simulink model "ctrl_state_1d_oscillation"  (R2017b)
settings: Solver=ode45  StartTime=0.0  StopTime=60  RelTol=1e-3
undefined symbols (not defined in the file or in its folder): b
libraries: dps x8

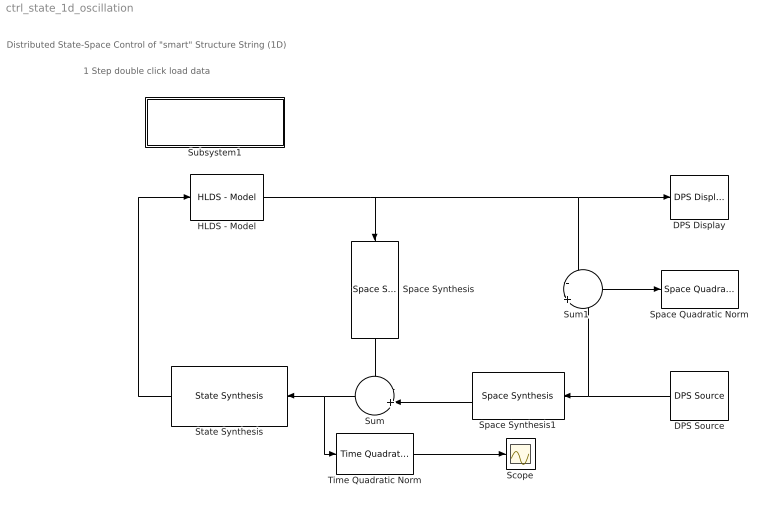
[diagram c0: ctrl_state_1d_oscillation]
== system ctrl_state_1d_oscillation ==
  note: Distributed State-Space Control of "smart" Structure String (1D)
  note: 1 Step double click load data
  DPS Display : dps/DPS Display  graphType=surf  pointCoord=[0:10]'  elementsVar=[1 2; 2 3; 3 4; 4 5; 5 6; 6 7; 7 8; 8 9; 9 10; 10 11]  showColor=on  minC=0  maxC=6  showDeform=off  deform=z  deformScale=0.001  showScope=off  responseVar=H  aviparam=0
  DPS Source : dps/DPS Source  equation=[0;1.52662144108251;2.42840593203700;3.01398701211897;3.50742289264669;3.74292718773858;3.88045730974050;3.89932061505839;3.38526460975261;2.00280456273636;0.00000000000000]  responseVar=0  showInput=on  pointsCoord=[0:10]'  elementsVar=[1 2; 2 3; 3 4; 4 5; 5 6; 6 7; 7 8; 8 9; 9 10; 10 11]  samplePeriod=1
  HLDS - Model : dps/Controlled Systems/HLDS - Model  StepResponse=H  samplePeriod=1  u_step=1
  Scope : Scope
  Space Quadratic Norm : dps/Quadratic norms/Space Quadratic Norm  StepResponse=H  showNorm=on
  Space Synthesis : dps/Space Synthesis/Space Synthesis  PCH=H  weights=[]
  Space Synthesis1 : dps/Space Synthesis/Space Synthesis  PCH=H  weights=[]
  State Synthesis : dps/Temporal Synthesis/State Synthesis  b=b  a=a  Q=1e-3*[7 0.8 2 0.2 0.51]  R={2e7, 3e7, 1.5e7, 1.5e7}  SamplePeriod=1
  Subsystem1 : Subsystem
  Sum : Sum  Inputs=-+|
  Sum1 : Sum  Inputs=-|+
  Time Quadratic Norm : dps/Quadratic norms/Time Quadratic Norm
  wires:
  State Synthesis/1 -> HLDS - Model/1
  DPS Source/1 -> Sum1/2, Space Synthesis1/1
  HLDS - Model/1 -> Space Synthesis/1, Sum1/1, DPS Display/1
  Space Synthesis/1 -> Sum/1
  Space Synthesis1/1 -> Sum/2
  Sum/1 -> Time Quadratic Norm/1, State Synthesis/1
  Sum1/1 -> Space Quadratic Norm/1
  Time Quadratic Norm/1 -> Scope/1

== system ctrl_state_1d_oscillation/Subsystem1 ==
